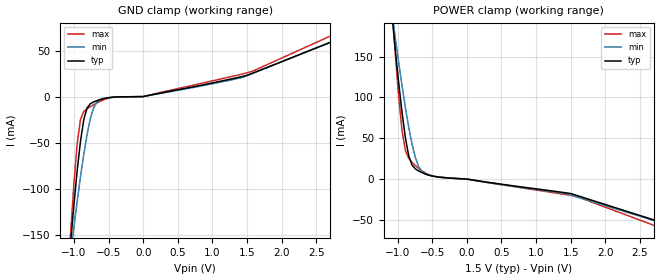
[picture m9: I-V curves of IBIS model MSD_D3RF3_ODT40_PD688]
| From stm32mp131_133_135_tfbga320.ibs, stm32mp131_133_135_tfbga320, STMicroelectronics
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[Model] MSD_D3RF3_ODT40_PD688
Model_type   Input
C_comp 2.343pF   2.301pF   2.421pF
Vinh = 925.000mV
Vinl = 575.000mV
[Model Spec]
Vinh   925.000mV   888.000mV   963.000mV
Vinl   575.000mV   538.000mV   613.000mV
[Temperature Range]   25.000   125.000   -40.000
[Voltage Range]   1.500V   1.425V   1.575V
[GND Clamp Reference]   0.00V   0.00V   0.00V
[POWER Clamp Reference]   1.500V   1.425V   1.575V
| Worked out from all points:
|   GND clamp passes 1 mA (typ) near -0.48 V on its own axis
|   POWER clamp passes 1 mA (typ) near -0.21 V on its own axis
[GND Clamp]
-1.48V    -590mA     -457.6mA   -789.2mA
-1.05V    -159.6mA   -172mA     -149.9mA
-1.002V   -118.2mA   -142.4mA   -95.4mA
-954.6mV  -80.76mA   -114mA     -51.31mA
-906.8mV  -48.84mA   -87.28mA   -25.02mA
-859.1mV  -25.11mA   -62.81mA   -16.32mA
-763.6mV  -7.714mA   -23.96mA   -10.91mA
-715.9mV  -5.76mA    -11.98mA   -8.8mA
-620.5mV  -3.292mA   -3.012mA   -5.046mA
900nV     14.18nA    13.04nA    16.65nA
1.575V    25.25mA    25.13mA    27.43mA
2.959V    66.72mA    66.42mA    74.47mA
[Power Clamp]
-1.459V   583.5mA    459.3mA    773mA
-1.077V   198mA      201.7mA    208.4mA
-1.03V    155.6mA    171.2mA    150.4mA
-981.8mV  116.3mA    141.7mA    98.53mA
-934.1mV  80.61mA    113.6mA    58.24mA
-886.4mV  50.24mA    87.29mA    34.97mA
-838.6mV  28.35mA    63.48mA    25.38mA
-790.9mV  17.17mA    42.85mA    20.5mA
-695.5mV  9.9mA      15.32mA    13.13mA
-504.6mV  3.79mA     3.912mA    4mA
1.548V    -19.01mA   -20.82mA   -20.65mA
2.98V     -57.59mA   -57.9mA    -65.41mA
